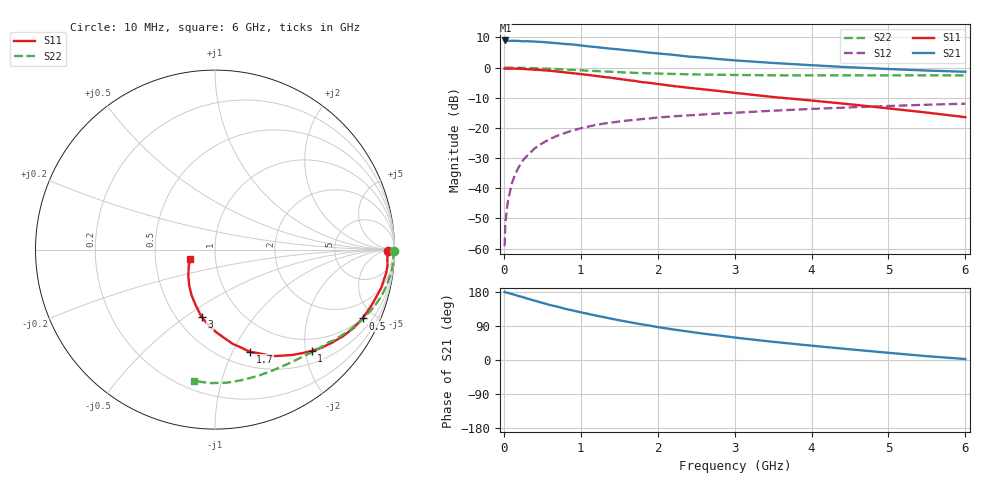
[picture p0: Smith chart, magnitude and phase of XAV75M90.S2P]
! SIEMENS Discrete & RF Semiconductors
! BFY180
! Si NPN RF Bipolar Junction Transistor in MICRO-X
! VCE = 0.75 V  IC = 0.9 mA
! Common Emitter S-Parameters:  May  1997
# GHz  S  MA  R  50
!  f  S11  S21  S12  S22
! GHz  MAG  ANG  MAG  ANG  MAG  ANG  MAG  ANG
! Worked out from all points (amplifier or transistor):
!   36 points, 10 MHz to 6 GHz, reference 50 ohm
!   highest |S21| = 9.0 dB at 20 MHz (marker M1)
!   |S21| within 3 dB of that: start of sweep to 1.51 GHz
!   unconditionally stable (mu >= 1): 2.941 GHz to end of sweep
!   at 250 MHz: K = 0.10, MSG = 19.7 dB, |S12| = -30.7 dB
!   at 1.4 GHz: K = 0.59, MSG = 12.2 dB, |S12| = -18.2 dB
!   at 6 GHz: K = 1.14, MAG = 3.0 dB, |S12| = -12.0 dB
!   S11 on the Smith chart (normalised r, x): 10 MHz: 53, -10; 500 MHz: 0.99, -4.30; 1 GHz: 0.74, -2.13; 1.7 GHz: 0.66, -1.17; 3 GHz: 0.66, -0.58; 6 GHz: 0.75, -0.08
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0.01  0.9644 -0.4  2.759 179.8  0.0011 86.8  0.9956 -0.3
0.02  0.962 -1.2  2.817 178.7  0.0027 94.7  0.999 -0.6
0.05  0.9612 -2.5  2.781 177.3  0.0058 85.6  0.9955 -1.5
0.1  0.9652 -5.1  2.777 174.4  0.0117 86.8  0.9947 -3.0
0.15  0.9629 -7.9  2.781 171.4  0.0174 84.9  0.9946 -4.4
0.25  0.9508 -12.9  2.728 165.7  0.0293 81.4  0.9905 -7.3
0.4  0.9244 -20.0  2.703 156.6  0.0458 76.0  0.9782 -11.5
0.5  0.9076 -25.0  2.653 150.9  0.0558 72.1  0.9673 -14.3
0.6  0.8867 -29.6  2.592 145.1  0.0658 69.2  0.9567 -16.8
0.8  0.8323 -38.6  2.459 134.9  0.0832 63.1  0.9293 -21.8
1  0.7801 -46.3  2.33 125.9  0.0987 57.4  0.9018 -26.4
1.1  0.7544 -49.9  2.251 121.6  0.1054 54.9  0.8884 -28.3
1.4  0.6779 -61.1  2.054 108.9  0.1229 48.5  0.852 -34.2
1.7  0.6022 -71.1  1.891 97.3  0.136 43.4  0.8181 -39.1
2  0.5357 -79.2  1.72 86.9  0.149 39.3  0.7987 -43.8
2.2  0.496 -83.9  1.629 80.7  0.1557 36.5  0.7859 -46.9
2.6  0.4355 -93.1  1.462 69.3  0.1674 32.5  0.7662 -52.3
3  0.3822 -101.3  1.318 59.3  0.1785 28.5  0.7545 -57.7
3.5  0.3258 -109.5  1.193 48.0  0.1932 24.7  0.7463 -64.2
4.5  0.2467 -125.6  1.013 28.2  0.2191 16.1  0.7426 -77.8
5.5  0.1797 -145.0  0.894 10.1  0.2426 7.6  0.7442 -92.1
6  0.1509 -159.4  0.853 2.5  0.2526 3.2  0.741 -99.3
